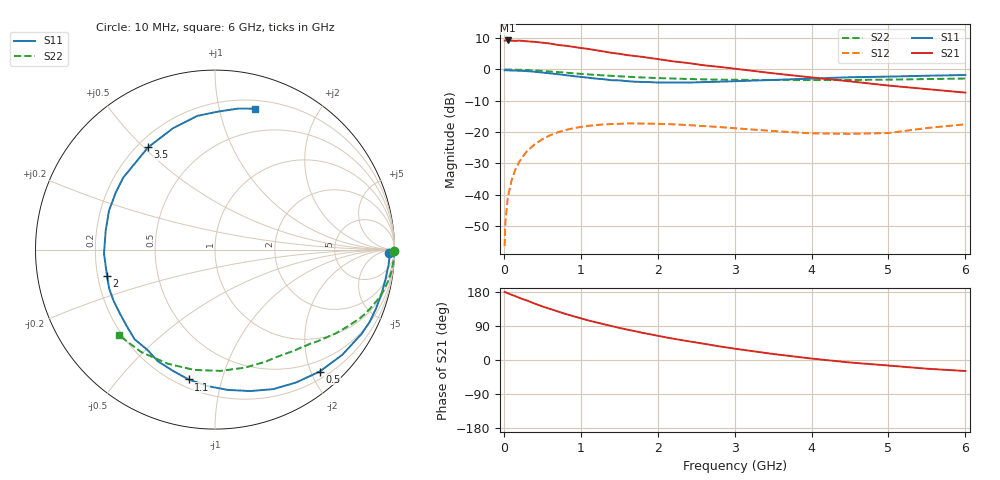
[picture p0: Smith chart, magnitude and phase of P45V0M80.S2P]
! SIEMENS Small Signal Semiconductors
! BFP182
! Si NPN RF Bipolar Junction Transistor in SOT143
! VCE = 5 V  IC = 0.8 mA
! Common Emitter S-Parameters:  March  1996
# GHz  S  MA  R  50
!  f  S11  S21  S12  S22
! GHz  MAG  ANG  MAG  ANG  MAG  ANG  MAG  ANG
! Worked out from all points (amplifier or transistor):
!   36 points, 10 MHz to 6 GHz, reference 50 ohm
!   highest |S21| = 9.3 dB at 50 MHz (marker M1)
!   |S21| within 3 dB of that: start of sweep to 1.168 GHz
!   unconditionally stable (mu >= 1): 2.773 GHz to end of sweep
!   at 250 MHz: K = 0.09, MSG = 18.4 dB, |S12| = -27.7 dB
!   at 1.4 GHz: K = 0.52, MSG = 11.4 dB, |S12| = -17.5 dB
!   at 6 GHz: K = 1.09, MAG = 3.3 dB, |S12| = -17.5 dB
!   S11 on the Smith chart (normalised r, x): 10 MHz: 50, -29; 500 MHz: 0.31, -2.14; 1.1 GHz: 0.25, -0.79; 2 GHz: 0.24, -0.11; 3.5 GHz: 0.24, +0.52; 6 GHz: 0.27, +1.29
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0.01  0.9702 -1.0  2.899 179.5  0.0015 96.9  0.9982 -0.4
0.02  0.9744 -2.0  2.902 179.1  0.0036 89.6  0.9928 -0.7
0.05  0.9706 -5.1  2.912 176.2  0.0087 88.4  0.9985 -1.8
0.1  0.964 -10.0  2.894 172.2  0.0168 82.2  0.9957 -3.7
0.2  0.9554 -20.2  2.898 164.2  0.0333 77.5  0.9897 -7.3
0.4  0.9201 -39.6  2.768 148.9  0.0636 65.0  0.9646 -14.2
0.5  0.8953 -49.4  2.685 141.4  0.0767 59.0  0.9466 -17.4
0.6  0.8673 -58.6  2.603 134.8  0.0887 53.4  0.9272 -20.4
0.8  0.8119 -76.1  2.398 121.7  0.1075 43.7  0.8908 -25.7
1.1  0.7381 -101.5  2.131 104.3  0.1258 30.7  0.8346 -32.5
1.3  0.6987 -117.1  1.941 94.4  0.1325 23.7  0.805 -36.4
1.5  0.6709 -131.9  1.784 84.8  0.1355 17.6  0.778 -39.9
1.8  0.6329 -153.3  1.592 71.8  0.1369 10.3  0.746 -44.6
2  0.6192 -166.3  1.469 63.9  0.1356 6.1  0.7288 -47.9
2.2  0.6188 -178.0  1.35 56.3  0.133 2.1  0.7177 -51.3
2.8  0.6379 150.1  1.102 36.0  0.1204 -5.2  0.6878 -61.6
3.5  0.6809 123.2  0.87 15.9  0.1039 -7.1  0.6785 -75.7
4  0.7156 109.1  0.747 3.8  0.0954 -2.6  0.6764 -87.3
4.5  0.7516 97.5  0.646 -6.6  0.0937 3.5  0.6803 -99.7
5  0.7693 88.6  0.554 -14.6  0.0965 13.3  0.6881 -112.4
5.5  0.7953 80.9  0.486 -23.0  0.116 16.1  0.7035 -125.7
6  0.8159 74.2  0.427 -29.0  0.1331 15.9  0.7175 -138.4
